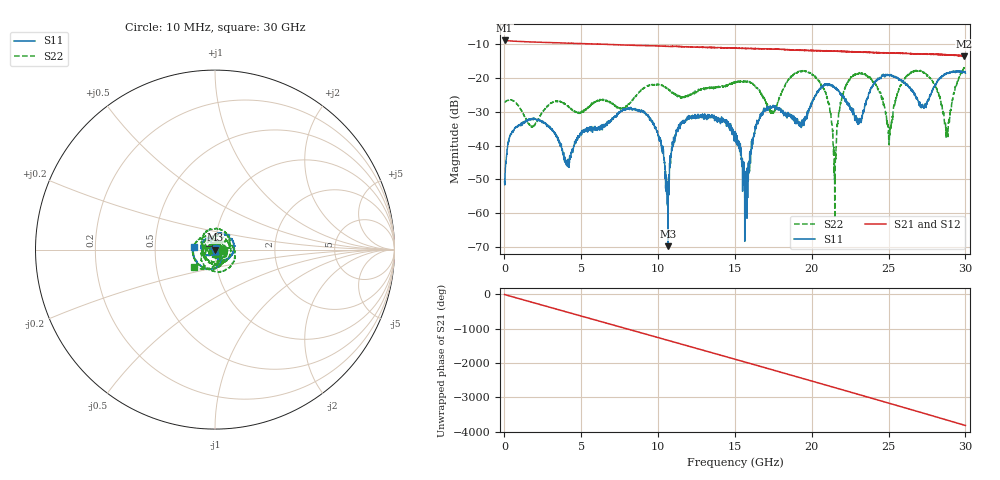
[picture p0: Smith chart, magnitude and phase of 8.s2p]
#  HZ  S  DB  R  50.00
! Rohde & Schwarz Vector Network Analyzer
! Rohde-Schwarz,ZNB40-4Port,1311601084101679,3.45
! Created: UTC 10/20/2022, 5:24:16 PM
! freq[Hz]  db:S11  ang:S11  db:S31  ang:S31  db:S13  ang:S13  db:S33  ang:S33
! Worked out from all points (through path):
!   3000 points, 10 MHz to 30 GHz, reference 50 ohm
!   highest |S21| = -8.93 dB at 10 MHz (marker M1); lowest = -13.6 dB at 29.94 GHz (marker M2)
!   group delay of S21, straight-line fit = 353 ps
!   lowest |S11| = -69.7 dB at 10.65 GHz (marker M3), VSWR 1.00, Z = 50 - j0.0229 ohm
!   |S11| at or under -10 dB: start of sweep to end of sweep
!   |S22| runs from -61.4 to -16.4 dB; largest |S21 - S12| = 0.007
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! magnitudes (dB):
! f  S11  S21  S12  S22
! 10 MHz  -50.7  -8.9  -8.9  -27.1
! 400 MHz  -36.6  -9.1  -9.1  -26.5
! 1.5 GHz  -32.5  -9.3  -9.3  -32.8
! 4.07 GHz  -45.6  -9.7  -9.7  -28.2
! 5.01 GHz  -36.2  -9.9  -9.9  -30.1
! 8.11 GHz  -29.0  -10.3  -10.3  -27.7
! 10.01 GHz  -36.9  -10.6  -10.6  -22.1
! 10.65 GHz  -69.7  -10.7  -10.7  -23.3
! 11.93 GHz  -31.5  -10.8  -10.8  -25.6
! 15.01 GHz  -37.4  -11.2  -11.2  -21.4
! 15.74 GHz  -49.7  -11.3  -11.3  -21.1
! 16.83 GHz  -30.3  -11.4  -11.4  -25.6
! 20.01 GHz  -27.5  -11.8  -11.9  -18.8
! 21.01 GHz  -21.9  -12.0  -12.1  -26.1
! 21.49 GHz  -22.7  -12.1  -12.1  -48.8
! 21.99 GHz  -25.4  -12.2  -12.2  -25.0
! 22.79 GHz  -31.6  -12.3  -12.3  -19.1
! 25.01 GHz  -19.2  -12.7  -12.6  -38.3
! 26.84 GHz  -26.0  -12.9  -12.9  -17.9
! 28.81 GHz  -18.5  -13.2  -13.1  -34.8
! 29.94 GHz  -18.2  -13.6  -13.5  -16.9
! 30 GHz  -18.6  -13.5  -13.5  -16.4
